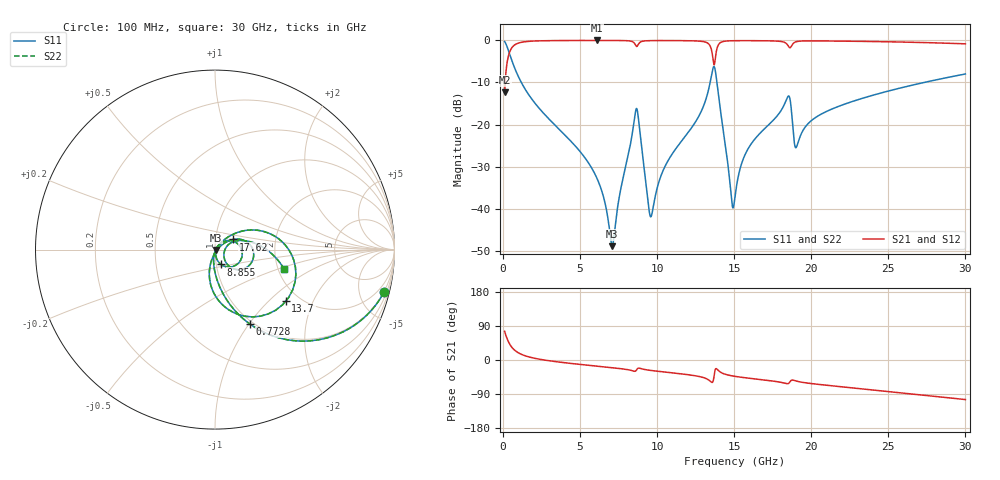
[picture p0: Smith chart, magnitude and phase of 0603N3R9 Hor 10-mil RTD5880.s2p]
# GHz S MA R 50
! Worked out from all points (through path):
!   3201 points, 100 MHz to 30 GHz, reference 50 ohm
!   highest |S21| = -0.03 dB at 6.08 GHz (marker M1); lowest = -12.4 dB at 100 MHz (marker M2)
!   group delay of S21, straight-line fit = 10.7 ps
!   lowest |S11| = -48.9 dB at 7.08 GHz (marker M3), VSWR 1.01, Z = 50.3 - j0.149 ohm
!   |S11| at or under -10 dB: 1.185 GHz to 13.44 GHz (12.25 GHz wide, 168 % of centre); 13.88 GHz to 27.32 GHz (13.44 GHz wide, 65.3 % of centre)
!   |S22| runs from -48.9 to -0.3 dB; largest |S21 - S12| = 0
!   S11 on the Smith chart (normalised r, x): 100 MHz: 0.96, -7.91; 772.8 MHz: 0.96, -1.01; 8.855 GHz: 1.05, -0.18; 13.7 GHz: 1.69, -1.28; 17.62 GHz: 1.22, +0.14; 30 GHz: 2.15, -0.55
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0.1  0.9706 -14.2  0.2406 75.8  0.2406 75.8  0.9706 -14.2
0.3803125  0.7267 -44.5  0.6865 45.5  0.6865 45.5  0.7267 -44.5
0.77275  0.4594 -64.8  0.8874 25.1  0.8874 25.1  0.4594 -64.8
5.089563  0.04559 -99.1  0.9965 -12.1  0.9965 -12.1  0.04559 -99.1
6.08  0.02331 -99.3  0.9969 -16.2  0.9969 -16.2  0.02331 -99.3
7.079781  0.003604 -24.3  0.9963 -20.3  0.9963 -20.3  0.003604 -24.3
8.565437  0.1326 13.1  0.8985 -29.8  0.8985 -29.8  0.1326 13.1
8.855094  0.08901 -68.1  0.9364 -21.7  0.9364 -21.7  0.08901 -68.1
9.527844  0.008438 -34.3  0.9915 -27.2  0.9915 -27.2  0.008438 -34.3
10.06978  0.01968 42.7  0.9938 -29.9  0.9938 -29.9  0.01968 42.7
13.29337  0.2421 26.9  0.9224 -51.5  0.9224 -51.5  0.2421 26.9
13.69516  0.4885 -36.2  0.5124 -41.5  0.5124 -41.5  0.4885 -36.2
14.03153  0.1864 -98.2  0.916 -29.8  0.916 -29.8  0.1864 -98.2
14.82575  0.01278 -71.3  0.9887 -41.6  0.9887 -41.6  0.01278 -71.3
15.05  0.01383 5.1  0.9905 -43.2  0.9905 -43.2  0.01383 5.1
15.7975  0.04772 34.4  0.9918 -47.3  0.9918 -47.3  0.04772 34.4
17.61953  0.1171 28.7  0.9826 -56.2  0.9826 -56.2  0.1171 28.7
18.52587  0.2187 -11.0  0.8467 -61.6  0.8467 -61.6  0.2187 -11.0
19.03044  0.05386 -5.6  0.9643 -55.6  0.9643 -55.6  0.05386 -5.6
20.03956  0.1128 23.3  0.9848 -62.4  0.9848 -62.4  0.1128 23.3
25.01978  0.2507 5.3  0.9611 -83.2  0.9611 -83.2  0.2507 5.3
30  0.3988 -15.5  0.9091 -104.4  0.9091 -104.4  0.3988 -15.5
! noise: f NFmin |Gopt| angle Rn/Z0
0.1  0.000364  0.9352  0.8183  0.001251
3.417  0.003758  0.7974  10.01  0.003809
6.743  0.006872  0.7841  19.42  0.006355
10.06  0.01133  0.8041  28.76  0.01128
13.39  0.04858  0.9355  37.99  0.1501
16.7  0.01559  0.7733  46.9  0.01185
20.03  0.01903  0.7798  55.67  0.01391
23.35  0.0178  0.7364  63.87  0.00981
26.67  0.01988  0.735  71.94  0.009939
30  0.0224  0.7393  79.76  0.01029
